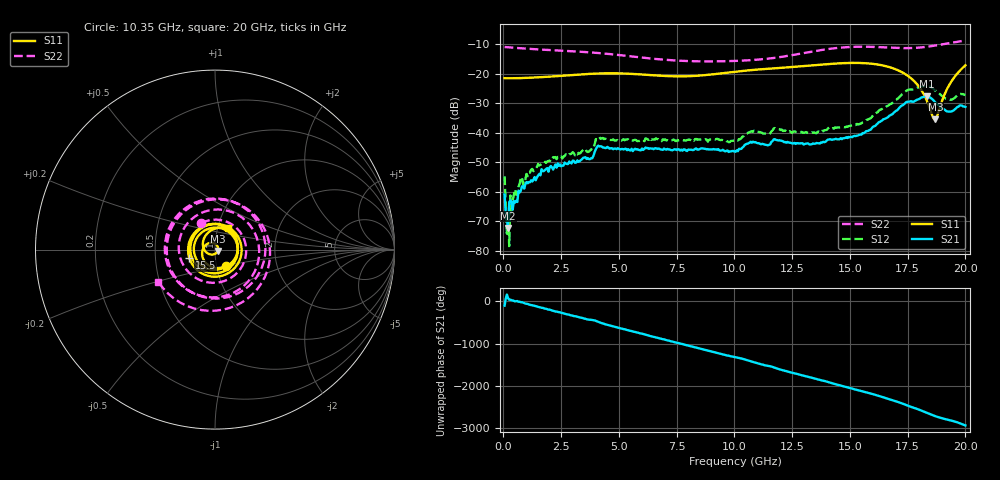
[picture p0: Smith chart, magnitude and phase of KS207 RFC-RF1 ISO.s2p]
!Agilent	"Technologies,E8364B,MY43040668,A.07.50.67"
!Agilent	E8364B:	A.07.50.67
!Date:	"Friday,"	June	"03,"	2022	13:36:14
!Correction:	S11(Full	2	"Port(1,2))"
!S21(Full	2	"Port(1,2))"
!S12(Full	2	"Port(1,2))"
!S22(Full	2	"Port(1,2))"
!S2P	File:	Measurements:	"S11,"	"S21,"	"S12,"	S22:
#	Hz	S	dB	R	50
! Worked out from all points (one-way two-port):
!   400 points, 50 MHz to 20 GHz, reference 50 ohm
!   highest |S21| = -27.71 dB at 18.35 GHz (marker M1); lowest = -72.2 dB at 200 MHz (marker M2)
!   lowest |S11| = -35.5 dB at 18.7 GHz (marker M3), VSWR 1.03, Z = 51.5 - j0.858 ohm
!   |S11| at or under -10 dB: start of sweep to end of sweep
!   |S22| runs from -15.9 to -8.8 dB; largest |S21 - S12| = 0.022
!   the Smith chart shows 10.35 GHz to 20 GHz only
!   S11 on the Smith chart (normalised r, x): 10.35 GHz: 1.11, -0.21; 15.5 GHz: 0.75, -0.07; 20 GHz: 1.12, +0.27
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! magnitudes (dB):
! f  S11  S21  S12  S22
! 50 MHz  -21.6  -61.0  -54.8  -11.0
! 150 MHz  -21.6  -69.1  -74.2  -11.1
! 200 MHz  -21.6  -72.2  -67.9  -11.1
! 250 MHz  -21.6  -63.5  -78.4  -11.1
! 300 MHz  -21.6  -62.9  -61.3  -11.2
! 350 MHz  -21.6  -63.5  -67.2  -11.2
! 500 MHz  -21.6  -63.7  -59.2  -11.3
! 750 MHz  -21.5  -59.7  -55.2  -11.4
! 1.65 GHz  -21.2  -52.4  -50.6  -11.9
! 3.4 GHz  -20.3  -49.0  -46.2  -12.7
! 4.15 GHz  -20.0  -44.7  -41.4  -13.1
! 6.7 GHz  -20.7  -45.4  -42.2  -15.1
! 10.05 GHz  -19.4  -46.5  -42.7  -15.7
! 10.35 GHz  -19.1  -45.0  -41.3  -15.6
! 13.35 GHz  -17.2  -43.9  -39.9  -12.6
! 15.5 GHz  -16.4  -40.7  -36.8  -10.9
! 16.7 GHz  -17.8  -34.3  -30.6  -11.2
! 17.7 GHz  -22.0  -29.5  -25.4  -11.4
! 18.35 GHz  -29.5  -27.7  -24.2  -10.9
! 18.7 GHz  -35.5  -29.8  -25.8  -10.5
! 19.3 GHz  -23.9  -32.9  -28.7  -9.7
! 20 GHz  -17.2  -31.3  -27.2  -8.8
